(* Logix 5000 AddOnInstructionDefinition export YAI_Assy_151_20_21_EIP_Hz; software revision 17.00 *)

ADD_ON_INSTRUCTION YAI_Assy_151_20_21_EIP_Hz   (* revision 1.0, vendor Yaskawa America, Inc. *)
// YAI Assembly 151 and 20/21
// Help:
// This add-on instruction is for use with input assembly 151 and output assemblies 20 or 21.
// Node_Input_Assy is defined as the node's input assembly integer array.
// Node_Output_Assy is defined as the node's output assembly integer array.
VAR_IN_OUT
   Node_Input_Assy : AB:ETHERNET_MODULE_INT_8Bytes:I:0; {required}   // Input assembly words
   Node_Output_Assy : AB:ETHERNET_MODULE_INT_4Bytes:O:0; {required}   // Output assembly words
END_VAR
VAR_INPUT
   RunFwd : BOOL; {visible}   // Forward run command
   RunRev : BOOL; {visible}   // Reverse run command
   FaultReset : BOOL; {visible}   // Fault reset command
   Net_Control : BOOL;   // Network control bit to switch between b1-02 setting and network.
   Net_Ref : BOOL;   // Network reference bit to switch between b1-01 setting and network.
   Freq_Ref : REAL; {visible}   // Frequency reference command in Hz (xx.xx resolution)
END_VAR
VAR_OUTPUT
   Faulted : BOOL; {visible}   // Drive faulted status bit
   Alarm : BOOL; {visible}   // Drive warning (alarm) status bit
   Ready : BOOL; {visible}   // Drive ready status bit
   NetRefStatus : BOOL; {visible}   // Drive network reference status bit (1 = reference coming from network)
   NetCtrlStatus : BOOL; {visible}   // Drive network run source status bit (1 = source coming from network)
   At_Speed : BOOL; {visible}   // Drive at commanded speed status bit
   Output_Freq : REAL; {visible}   // Drive output frequency in Hz (xx.xx resolution)
   Running : BOOL; {visible}
   ZSP : BOOL;
   RunningRev : BOOL; {visible}
   Reset : BOOL;
   OPE : BOOL;
   UV : BOOL;
   MFO_1_Status : BOOL;
   MFO_2_Status : BOOL;
   MFO_3_Status : BOOL;
   ZSV : BOOL;
   Torque_Actual : REAL; {visible}
   Output_Current : REAL; {visible}
END_VAR
VAR
   FRef_Convert : DINT;
   FOut_Convert : REAL;
   FOut_Temp : REAL;
   Fault_Reset_Timer : TIMER := (PRE := 250);
   TOut_Temp : REAL;
   TOut_Convert : REAL;
   IOut_Temp : REAL;
   IOut_Convert : REAL;
END_VAR

ROUTINE Logic   (* ladder *)
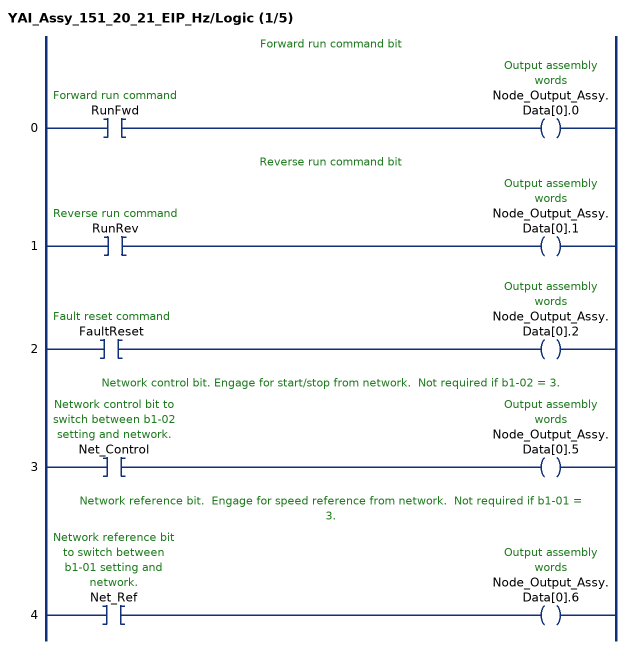
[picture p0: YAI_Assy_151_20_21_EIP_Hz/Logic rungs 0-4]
   // Forward run command bit
   0: XIC(RunFwd)OTE(Node_Output_Assy.Data[0].0);
   // Reverse run command bit
   1: XIC(RunRev)OTE(Node_Output_Assy.Data[0].1);
   2: XIC(FaultReset)OTE(Node_Output_Assy.Data[0].2);
   // Network control bit. Engage for start/stop from network.  Not required if b1-02 = 3.
   3: XIC(Net_Control)OTE(Node_Output_Assy.Data[0].5);
   // Network reference bit.  Engage for speed reference from network.  Not required if b1-01 = 3.
   4: XIC(Net_Ref)OTE(Node_Output_Assy.Data[0].6);
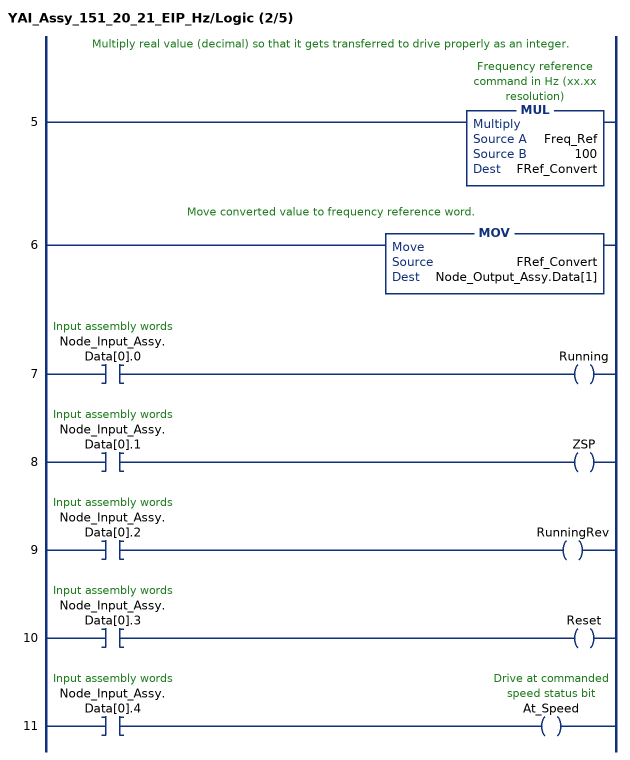
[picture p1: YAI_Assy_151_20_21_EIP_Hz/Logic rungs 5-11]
   // Multiply real value (decimal) so that it gets transferred to drive properly as an integer.
   5: MUL(Freq_Ref,100,FRef_Convert);
   // Move converted value to frequency reference word.
   6: MOV(FRef_Convert,Node_Output_Assy.Data[1]);
   7: XIC(Node_Input_Assy.Data[0].0)OTE(Running);
   8: XIC(Node_Input_Assy.Data[0].1)OTE(ZSP);
   9: XIC(Node_Input_Assy.Data[0].2)OTE(RunningRev);
   10: XIC(Node_Input_Assy.Data[0].3)OTE(Reset);
   11: XIC(Node_Input_Assy.Data[0].4)OTE(At_Speed);
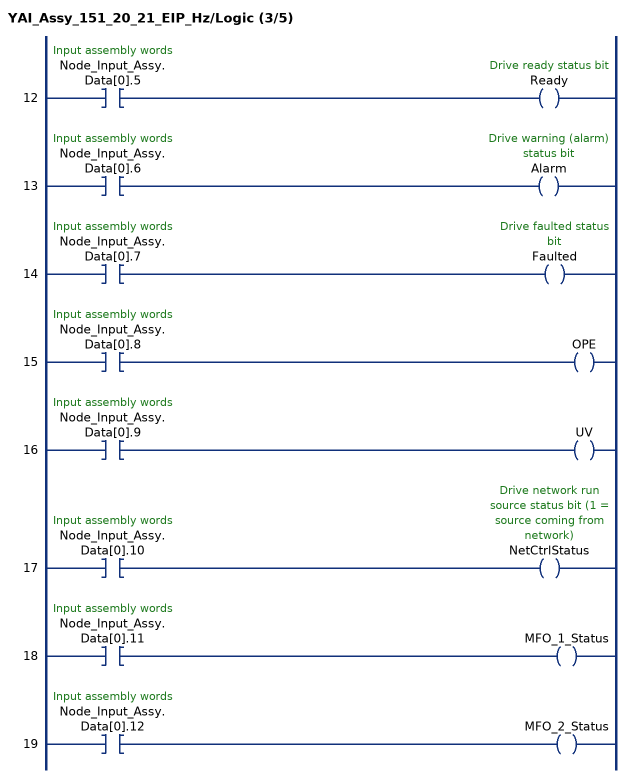
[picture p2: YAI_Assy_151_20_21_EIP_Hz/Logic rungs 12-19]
   12: XIC(Node_Input_Assy.Data[0].5)OTE(Ready);
   13: XIC(Node_Input_Assy.Data[0].6)OTE(Alarm);
   14: XIC(Node_Input_Assy.Data[0].7)OTE(Faulted);
   15: XIC(Node_Input_Assy.Data[0].8)OTE(OPE);
   16: XIC(Node_Input_Assy.Data[0].9)OTE(UV);
   17: XIC(Node_Input_Assy.Data[0].10)OTE(NetCtrlStatus);
   18: XIC(Node_Input_Assy.Data[0].11)OTE(MFO_1_Status);
   19: XIC(Node_Input_Assy.Data[0].12)OTE(MFO_2_Status);
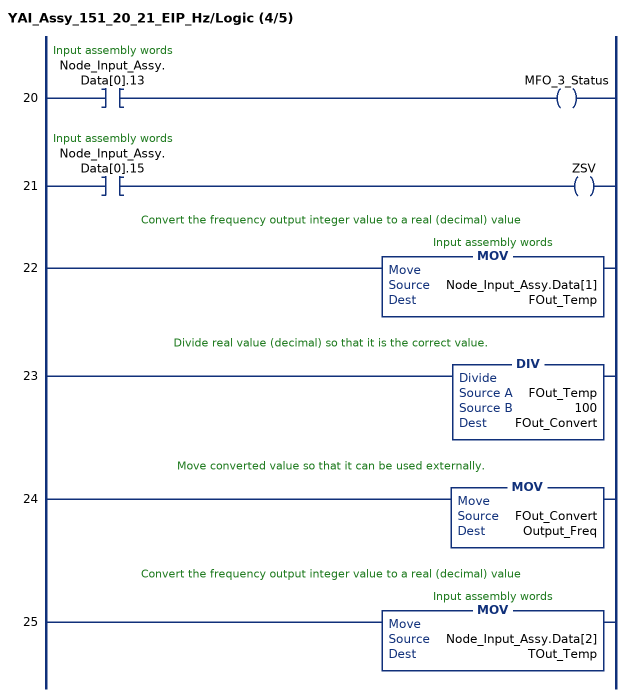
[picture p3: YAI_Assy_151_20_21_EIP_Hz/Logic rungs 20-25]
   20: XIC(Node_Input_Assy.Data[0].13)OTE(MFO_3_Status);
   21: XIC(Node_Input_Assy.Data[0].15)OTE(ZSV);
   // Convert the frequency output integer value to a real (decimal) value
   22: MOV(Node_Input_Assy.Data[1],FOut_Temp);
   // Divide real value (decimal) so that it is the correct value.
   23: DIV(FOut_Temp,100,FOut_Convert);
   // Move converted value so that it can be used externally.
   24: MOV(FOut_Convert,Output_Freq);
   // Convert the frequency output integer value to a real (decimal) value
   25: MOV(Node_Input_Assy.Data[2],TOut_Temp);
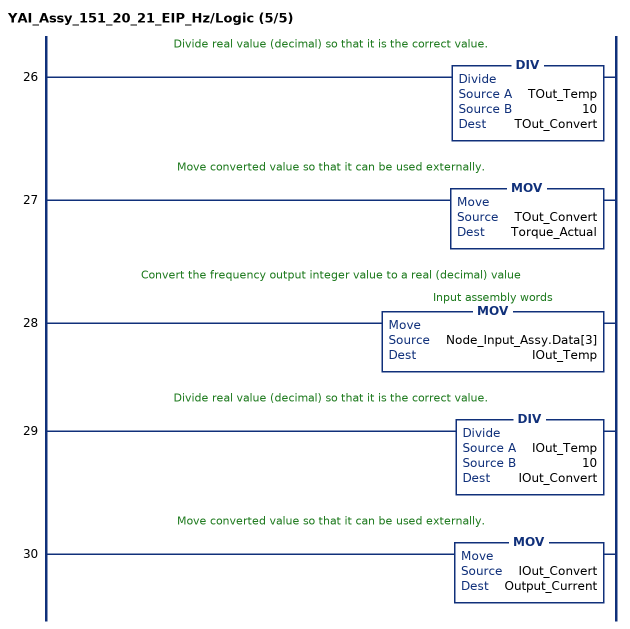
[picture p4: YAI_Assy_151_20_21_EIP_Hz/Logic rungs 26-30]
   // Divide real value (decimal) so that it is the correct value.
   26: DIV(TOut_Temp,10,TOut_Convert);
   // Move converted value so that it can be used externally.
   27: MOV(TOut_Convert,Torque_Actual);
   // Convert the frequency output integer value to a real (decimal) value
   28: MOV(Node_Input_Assy.Data[3],IOut_Temp);
   // Divide real value (decimal) so that it is the correct value.
   29: DIV(IOut_Temp,10,IOut_Convert);
   // Move converted value so that it can be used externally.
   30: MOV(IOut_Convert,Output_Current);
END_ROUTINE
END_ADD_ON_INSTRUCTION
